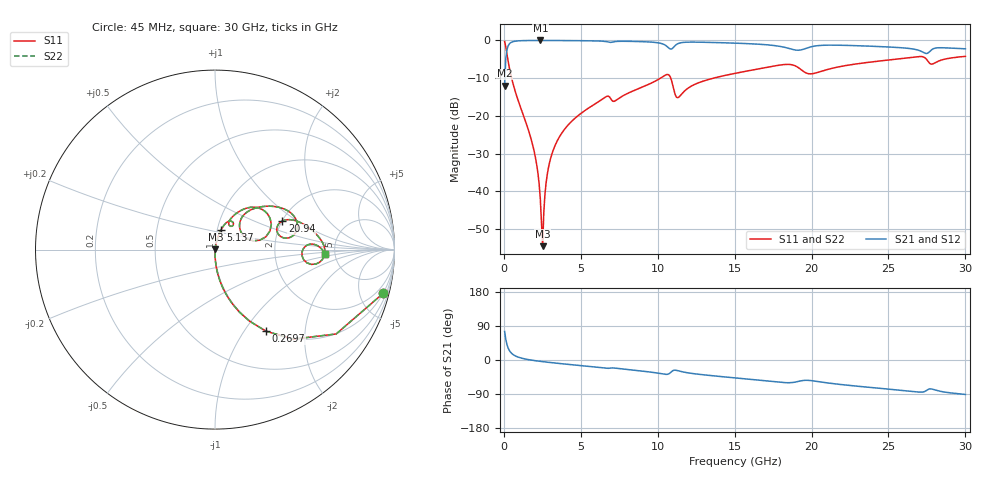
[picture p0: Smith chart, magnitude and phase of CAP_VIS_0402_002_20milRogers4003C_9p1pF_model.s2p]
! S-parameter model data by Modelithics Inc.  support@modelithics.com  813-866-6335  Tampa FL USA
! S-Parameter data specifications:
! Substrate: 20-mil Rogers 4003C, substrate thickness, H=0.508mm, Dielectric constant, Er=3.75
! PCB Mounting Pad Footprint: Pad width, PadW=0.50mm , Pad length, PadL=0.50mm , Pad gap, PadG (edge-to-edge)=0.40mm , Reference planes=1.4mm apart
! Created Wed Nov 18 12:50:27 2015
# hz S ma R 50
! 2 Port Network Data from SP1.SP block
! freq  magS11  angS11  magS21  angS21  magS12  angS12  magS22  angS22
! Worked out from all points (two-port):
!   401 points, 45 MHz to 30 GHz, reference 50 ohm
!   highest |S21| = -0.02 dB at 2.367 GHz (marker M1); lowest = -12.0 dB at 45 MHz (marker M2)
!   |S21| within 3 dB of the highest: 179.4 MHz to 27.19 GHz (27.01 GHz wide, 197 % of centre); 27.66 GHz to end of sweep
!   lowest |S11| = -54.5 dB at 2.516 GHz (marker M3), VSWR 1.00, Z = 50.2 + j0.064 ohm
!   |S11| at or under -10 dB: 501.1 MHz to 10.17 GHz (9.674 GHz wide, 181 % of centre); 10.85 GHz to 13.62 GHz (2.776 GHz wide, 22.7 % of centre)
!   |S22| runs from -54.5 to -0.3 dB; largest |S21 - S12| = 0
!   S11 on the Smith chart (normalised r, x): 45 MHz: 0.99, -7.69; 269.7 MHz: 0.99, -1.27; 5.137 GHz: 1.04, +0.23; 20.94 GHz: 2.00, +0.76; 30 GHz: 4.17, -0.30
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4.5e7  0.9681 -14.6  0.2505 75.4  0.2505 75.4  0.9681 -14.6
2.696625e8  0.5375 -57.9  0.8427 32.1  0.8427 32.1  0.5375 -57.9
6.441e8  0.2445 -76.7  0.9688 13.0  0.9688 13.0  0.2445 -76.7
1.917188e9  0.03761 -88.8  0.9977 -1.1  0.9977 -1.1  0.03761 -88.8
2.216738e9  0.01705 -87.4  0.9982 -2.8  0.9982 -2.8  0.01705 -87.4
2.366512e9  0.007991 -81.6  0.9982 -3.6  0.9982 -3.6  0.007991 -81.6
2.516288e9  0.001886 19.8  0.9982 -4.4  0.9982 -4.4  0.001886 19.8
2.890725e9  0.02039 78.7  0.9979 -6.1  0.9979 -6.1  0.02039 78.7
3.265162e9  0.03792 79.2  0.9972 -7.8  0.9972 -7.8  0.03792 79.2
5.062462e9  0.1101 73.6  0.991 -15.0  0.991 -15.0  0.1101 73.6
5.13735e9  0.1129 73.3  0.9906 -15.3  0.9906 -15.3  0.1129 73.3
1.007992e10  0.3077 49.9  0.925 -35.1  0.925 -35.1  0.3077 49.9
1.067902e10  0.353 29.5  0.8062 -37.2  0.8062 -37.2  0.353 29.5
1.135301e10  0.1764 36.5  0.9127 -28.7  0.9127 -28.7  0.1764 36.5
1.50225e10  0.3661 41.2  0.92 -47.2  0.92 -47.2  0.3661 41.2
1.86171e10  0.4795 16.9  0.7741 -59.9  0.7741 -59.9  0.4795 16.9
2.003996e10  0.3617 17.8  0.8294 -54.7  0.8294 -54.7  0.3617 17.8
2.093861e10  0.4068 23.0  0.8643 -60.0  0.8643 -60.0  0.4068 23.0
2.505742e10  0.5515 11.3  0.8172 -77.1  0.8172 -77.1  0.5515 11.3
2.745382e10  0.5681 -8.1  0.6708 -80.9  0.6708 -80.9  0.5681 -8.1
2.827759e10  0.5349 3.3  0.7994 -81.8  0.7994 -81.8  0.5349 3.3
3e10  0.6148 -2.1  0.7739 -90.9  0.7739 -90.9  0.6148 -2.1
